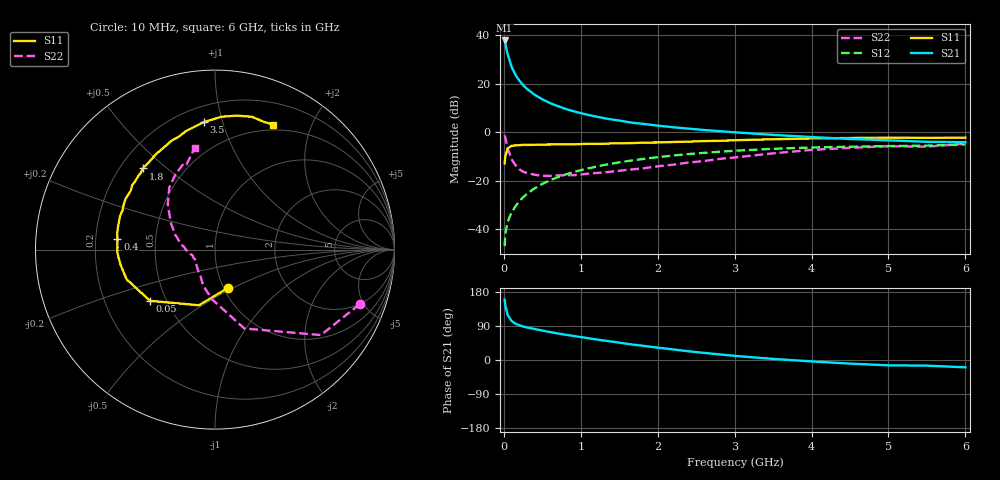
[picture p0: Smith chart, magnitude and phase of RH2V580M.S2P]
! SIEMENS Small Signal Semiconductors
! BFR106
! Si NPN RF Bipolar Junction Transistor in SOT23
! VCE = 2.5 V  IC = 80 mA
! Common Emitter S-Parameters:  August  1996
# GHz  S  MA  R  50
!  f  S11  S21  S12  S22
! GHz  MAG  ANG  MAG  ANG  MAG  ANG  MAG  ANG
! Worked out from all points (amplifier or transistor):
!   36 points, 10 MHz to 6 GHz, reference 50 ohm
!   highest |S21| = 37.9 dB at 10 MHz (marker M1)
!   |S21| within 3 dB of that: start of sweep to 31.3 MHz
!   unconditionally stable (mu >= 1): 176.1 MHz to 2.809 GHz; 5.193 GHz to end of sweep
!   at 250 MHz: K = 1.05, MAG = 21.8 dB, |S12| = -26.9 dB
!   at 1.4 GHz: K = 1.06, MAG = 7.6 dB, |S12| = -13.0 dB
!   at 6 GHz: K = 1.01, MAG = 0.0 dB, |S12| = -5.1 dB
!   S11 on the Smith chart (normalised r, x): 10 MHz: 1.04, -0.47; 50 MHz: 0.41, -0.29; 400 MHz: 0.29, +0.05; 1.8 GHz: 0.29, +0.42; 3.5 GHz: 0.30, +0.87; 6 GHz: 0.44, +1.48
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0.01  0.2263 -72.0  78.4 159.4  0.0044 78.1  0.8617 -20.7
0.02  0.3229 -106.1  67.21 143.7  0.0081 64.2  0.7581 -38.9
0.05  0.4611 -141.8  40.43 118.3  0.0142 60.8  0.469 -69.6
0.1  0.5199 -161.5  22.58 103.2  0.0217 65.4  0.2763 -93.7
0.15  0.5323 -170.5  15.38 96.0  0.0292 68.4  0.2089 -108.7
0.2  0.5381 -174.6  11.7 91.8  0.037 70.9  0.1718 -117.5
0.25  0.545 -178.6  9.363 88.5  0.045 71.8  0.152 -127.1
0.3  0.5434 178.9  7.836 86.0  0.053 72.6  0.144 -132.9
0.4  0.5473 173.8  5.929 81.8  0.069 73.2  0.1315 -142.9
0.5  0.5524 170.6  4.764 77.7  0.085 72.8  0.1252 -149.8
0.6  0.5554 166.5  3.991 73.8  0.1012 71.8  0.1246 -154.2
0.7  0.5579 163.1  3.452 70.1  0.117 70.9  0.1274 -158.1
0.9  0.5596 157.1  2.718 63.6  0.1485 67.9  0.1285 -165.5
1.1  0.5733 150.4  2.265 57.3  0.1786 64.9  0.1387 -169.8
1.4  0.5847 142.1  1.828 48.7  0.2228 60.0  0.1527 -176.7
1.8  0.6047 131.6  1.488 37.8  0.2777 53.3  0.1772 174.1
2.2  0.6251 121.8  1.262 27.9  0.3285 46.6  0.212 164.7
2.8  0.6606 107.8  1.05 14.9  0.393 36.6  0.2791 150.5
3.5  0.7129 95.0  0.878 2.9  0.4525 25.6  0.3642 136.2
4.5  0.7564 80.6  0.722 -9.6  0.5001 11.3  0.4742 117.6
5.5  0.762 69.0  0.632 -14.9  0.5265 2.4  0.5002 108.4
6  0.7681 64.9  0.62 -19.3  0.5557 -4.4  0.5783 101.3
